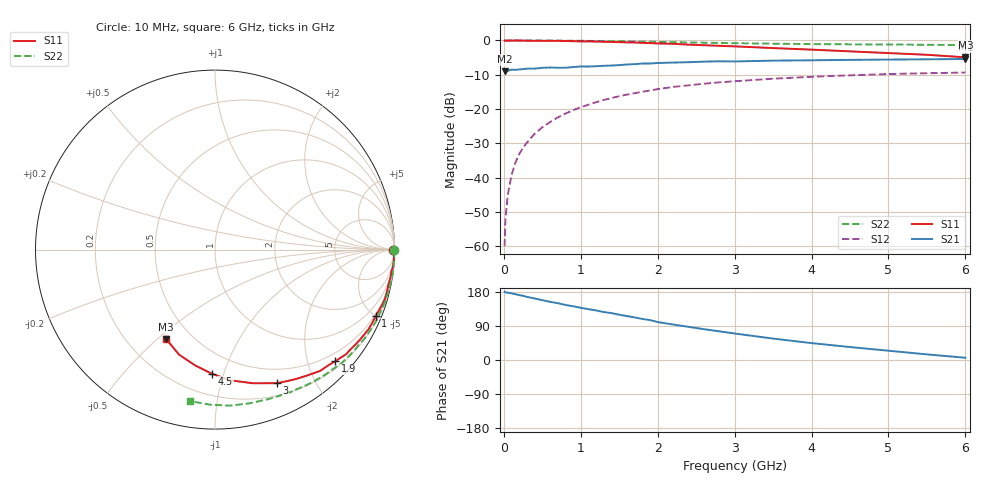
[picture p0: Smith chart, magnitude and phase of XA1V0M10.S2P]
! SIEMENS Discrete & RF Semiconductors
! BFY180
! Si NPN RF Bipolar Junction Transistor in MICRO-X
! VCE = 1 V  IC = 0.1 mA
! Common Emitter S-Parameters:  May  1997
# GHz  S  MA  R  50
!  f  S11  S21  S12  S22
! GHz  MAG  ANG  MAG  ANG  MAG  ANG  MAG  ANG
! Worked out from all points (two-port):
!   36 points, 10 MHz to 6 GHz, reference 50 ohm
!   highest |S21| = -5.42 dB at 6 GHz (marker M1); lowest = -9.0 dB at 10 MHz (marker M2)
!   |S21| within 3 dB of the highest: 218.3 MHz to end of sweep
!   lowest |S11| = -4.9 dB at 6 GHz (marker M3), VSWR 3.62, Z = 18.2 - j26.7 ohm
!   |S11| at or under -10 dB: nowhere
!   |S22| runs from -1.4 to 0.0 dB; largest |S21 - S12| = 0.39
!   S11 on the Smith chart (normalised r, x): 10 MHz: open; 1 GHz: 0.42, -5.02; 1.9 GHz: 0.33, -2.51; 3 GHz: 0.33, -1.51; 4.5 GHz: 0.34, -0.92; 6 GHz: 0.36, -0.53
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0.01  0.9945 -0.2  0.353 180.0  0.001 93.3  0.9999 -0.2
0.02  0.9847 -0.5  0.36 178.6  0.0024 93.3  0.9999 -0.4
0.05  0.9942 -1.1  0.36 177.7  0.0055 85.4  0.9989 -0.9
0.1  0.997 -2.2  0.376 176.0  0.0109 90.3  0.9992 -2.0
0.15  0.9985 -3.3  0.372 173.6  0.0166 88.2  0.9999 -3.0
0.2  0.9967 -4.5  0.378 171.2  0.0219 87.1  0.9992 -4.0
0.25  0.9953 -5.8  0.382 169.4  0.0274 85.3  0.9999 -5.0
0.3  0.9903 -7.0  0.388 166.5  0.0324 83.8  0.9979 -5.9
0.4  0.9902 -9.0  0.388 162.4  0.0435 82.1  0.9991 -7.8
0.5  0.986 -11.4  0.399 157.9  0.0542 79.6  0.9966 -9.9
0.7  0.9863 -16.1  0.4 150.0  0.0752 75.3  0.9939 -13.8
1  0.9687 -22.4  0.418 137.7  0.1062 68.7  0.9875 -19.8
1.1  0.9671 -24.7  0.417 134.3  0.1156 66.8  0.9834 -21.7
1.5  0.945 -33.9  0.437 119.5  0.1539 58.3  0.9718 -29.4
1.9  0.9149 -42.8  0.461 105.3  0.1863 50.5  0.9559 -36.8
2.2  0.8938 -49.2  0.476 93.7  0.2099 44.5  0.9461 -42.3
2.6  0.852 -57.6  0.491 81.4  0.2338 37.4  0.9279 -49.0
3  0.8198 -65.2  0.494 69.9  0.2541 30.4  0.9117 -55.5
3.5  0.7744 -74.1  0.508 56.5  0.277 23.1  0.8972 -62.8
4.5  0.6933 -91.2  0.521 34.2  0.31 8.9  0.8777 -77.4
5.5  0.618 -109.0  0.531 14.8  0.333 -4.4  0.8643 -92.1
6  0.5675 -118.7  0.536 5.9  0.3405 -11.1  0.8554 -99.4
